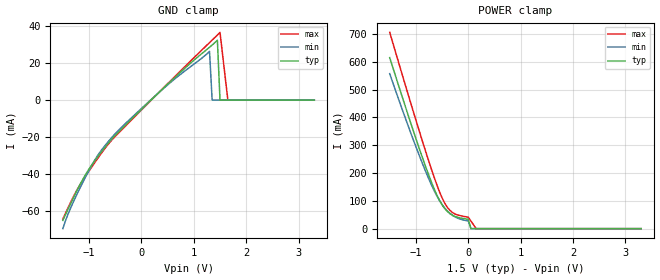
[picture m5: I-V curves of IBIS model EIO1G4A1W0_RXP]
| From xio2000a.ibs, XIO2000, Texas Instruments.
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|   Model EIO1G4A1W0_RXP
[Model]   EIO1G4A1W0_RXP
Model_type   Input
Polarity   Non-Inverting
Vinl =  -0.6000V
Vinh =   0.6000V
C_comp   1.6030pF   1.6370pF   1.5940pF
[Model Spec]
|   typ   min   max
Vinh   0.5V   0.175V   0.6V
Vinl   -0.5V   -0.175V   -0.6V
[Temperature Range]   25.0000   0.1250k   -40.0000
[Voltage Range]   1.5000V   1.3500V   1.6500V
[GND_clamp]
| voltage   I(typ)   I(min)   I(max)
-1.5V     -64.85mA   -69.3mA    -64.12mA
-1.35V    -55.75mA   -58.06mA   -55.04mA
-1.15V    -44.37mA   -46.09mA   -44.62mA
-750mV    -27.4mA    -26.47mA   -28.1mA
-400mV    -16.09mA   -15.2mA    -16.69mA
600mV     11.22mA    10.56mA    11.63mA
1.3V      28.48mA    26.24mA    30.98mA
1.35V     29.68mA    0A         32.34mA
1.45V     32.25mA    0A         35.08mA
1.5V      0A         0A         36.49mA
1.65V     0A         0A         0A
3.3V      0A         0A         0A
[POWER_clamp]
| voltage   I(typ)   I(min)   I(max)
-1.5V     614.8mA    557.3mA    705.6mA
-1.05V    352.1mA    319.6mA    421.1mA
-850mV    241.6mA    222.2mA    298.9mA
-700mV    165.3mA    155.9mA    211.5mA
-600mV    120.8mA    117.7mA    157.4mA
-500mV    85.47mA    86.47mA    110.5mA
-400mV    61.88mA    63.51mA    76.74mA
-300mV    47.9mA     47.74mA    57.86mA
0V        33.63mA    27.67mA    41.13mA
50mV      0A         0A         27.42mA
150mV     0A         0A         0A
3.3V      0A         0A         0A
